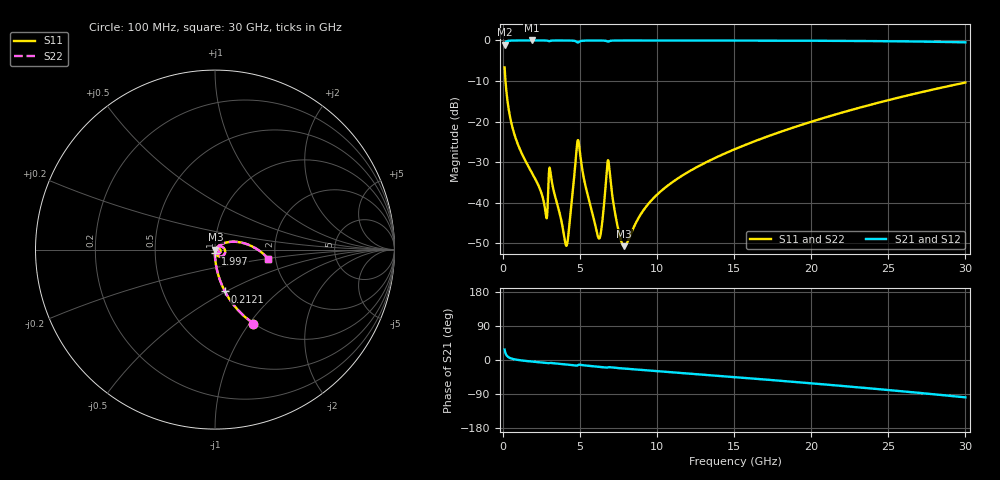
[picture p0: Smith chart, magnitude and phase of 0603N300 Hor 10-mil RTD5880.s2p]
# GHz S MA R 50
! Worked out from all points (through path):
!   3201 points, 100 MHz to 30 GHz, reference 50 ohm
!   highest |S21| = -0.01 dB at 1.857 GHz (marker M1); lowest = -1.1 dB at 100 MHz (marker M2)
!   group delay of S21, straight-line fit = 9.23 ps
!   lowest |S11| = -50.7 dB at 7.865 GHz (marker M3), VSWR 1.01, Z = 50.3 - j0.0942 ohm
!   |S11| at or under -10 dB: 157.2 MHz to end of sweep
!   |S22| runs from -50.7 to -6.7 dB; largest |S21 - S12| = 0
!   S11 on the Smith chart (normalised r, x): 100 MHz: 1.00, -1.05; 212.1 MHz: 1.00, -0.49; 1.997 GHz: 1.00, -0.04; 30 GHz: 1.83, -0.21
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0.1  0.4644 -62.6  0.8853 27.4  0.8853 27.4  0.4644 -62.6
0.212125  0.2396 -76.7  0.9705 13.3  0.9705 13.3  0.2396 -76.7
0.735375  0.06956 -87.5  0.9968 1.9  0.9968 1.9  0.06956 -87.5
1.856625  0.02364 -91.1  0.9985 -4.0  0.9985 -4.0  0.02364 -91.1
1.996781  0.02114 -91.1  0.9985 -4.6  0.9985 -4.6  0.02114 -91.1
2.753625  0.007655 -73.0  0.9968 -7.6  0.9968 -7.6  0.007655 -73.0
3.108687  0.02135 -74.9  0.9914 -7.9  0.9914 -7.9  0.02135 -74.9
4.099125  0.002942 -24.4  0.9971 -11.8  0.9971 -11.8  0.002942 -24.4
4.276656  0.004756 27.2  0.9963 -12.5  0.9963 -12.5  0.004756 27.2
4.799906  0.05189 6.5  0.9514 -14.9  0.9514 -14.9  0.05189 6.5
5.089563  0.0296 -75.5  0.9858 -13.2  0.9858 -13.2  0.0296 -75.5
6.210813  0.003635 -31.2  0.9964 -17.8  0.9964 -17.8  0.003635 -31.2
6.379  0.004702 8.9  0.9957 -18.5  0.9957 -18.5  0.004702 8.9
6.715375  0.02294 14.9  0.981 -20.1  0.981 -20.1  0.02294 14.9
6.855531  0.03098 -44.9  0.9719 -19.0  0.9719 -19.0  0.03098 -44.9
7.416156  0.005289 -70.4  0.9964 -21.1  0.9964 -21.1  0.005289 -70.4
7.864656  0.002915 -18.7  0.997 -22.6  0.997 -22.6  0.002915 -18.7
10.06978  0.01297 47.6  0.9969 -29.5  0.9969 -29.5  0.01297 47.6
15.05  0.04579 40.3  0.9952 -45.2  0.9952 -45.2  0.04579 40.3
20.03956  0.1 25.8  0.9903 -61.7  0.9903 -61.7  0.1 25.8
25.01978  0.184 9.0  0.9772 -79.3  0.9772 -79.3  0.184 9.0
30  0.3025 -9.8  0.9463 -98.6  0.9463 -98.6  0.3025 -9.8
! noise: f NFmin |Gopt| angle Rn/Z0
0.1  0.0002971  0.9198  0.3946  0.0008185
3.417  0.004423  0.8252  9.885  0.005276
6.743  0.01884  0.9154  19.41  0.04774
10.06  0.007958  0.7323  28.76  0.005572
13.39  0.009831  0.7173  37.94  0.006169
16.7  0.01175  0.71  46.86  0.006751
20.03  0.01373  0.7072  55.54  0.007275
23.35  0.0158  0.7078  63.93  0.007739
26.67  0.018  0.7112  72.06  0.008154
30  0.02039  0.7168  79.92  0.008521
